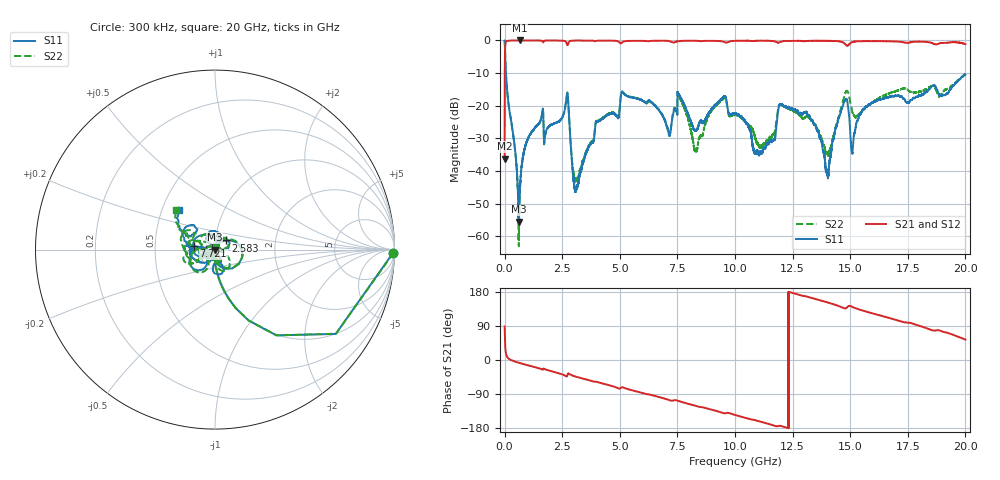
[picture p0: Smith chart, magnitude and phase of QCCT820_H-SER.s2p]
!{QCCT820}
!Johanson Technology Inc.
!www.johansontechnology.com
!Test Board Conditions:
!Substrate Type  RO4350B
!Substrate Thickness  20 mil
!Substrate Dk  3.66
!TL Type: GCPW
!TL Trace Width  34 mil
!TL Gap  10 mil
!Electrode orientation  Horizontal
!DUT TOPOLOGY	SERIES
!Mounting Pad LxW  26x52 mil
! Created Sat Jan  9 19:21:07 2021
# hz S ma R 50
! 2 Port Network Data from SP1.SP block
! freq  magS11  angS11  magS21  angS21  magS12  angS12  magS22  angS22
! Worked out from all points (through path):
!   20001 points, 300 kHz to 20 GHz, reference 50 ohm
!   highest |S21| = 0.00 dB at 661.3 MHz (marker M1); lowest = -36.2 dB at 300 kHz (marker M2)
!   group delay of S21, straight-line fit = 42 ps
!   lowest |S11| = -55.6 dB at 616.3 MHz (marker M3), VSWR 1.00, Z = 49.8 + j0.028 ohm
!   |S11| at or under -10 dB: 57.01 MHz to end of sweep
!   |S22| runs from -63.0 to 0.0 dB; largest |S21 - S12| = 0.015
!   S11 on the Smith chart (normalised r, x): 300 kHz: open; 2.583 GHz: 1.12, +0.12; 7.721 GHz: 0.79, +0.03; 20 GHz: 0.61, +0.30
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300000  0.9935 -0.9  0.01552 88.4  0.01569 89.2  0.9945 -1.0
1.113e8  0.1658 -82.3  0.9851 8.2  0.9851 8.1  0.1665 -82.1
6.163e8  0.001668 170.3  0.9989 -7.3  0.9988 -7.3  0.0007043 -161.2
6.613e8  0.004868 99.8  0.9995 -8.1  0.9977 -8.1  0.004485 90.4
1.1063e9  0.03639 77.6  0.9988 -15.5  0.9983 -15.5  0.03631 73.8
2.5833e9  0.07857 40.5  0.9843 -39.9  0.9856 -39.8  0.07863 45.1
2.7443e9  0.1404 -48.7  0.8591 -36.7  0.8591 -36.7  0.1416 -44.7
3.0543e9  0.005208 -132.3  0.9961 -43.2  0.9961 -43.2  0.007195 -86.5
3.3343e9  0.01071 -160.5  0.9977 -48.0  0.9977 -48.0  0.01145 -105.8
5.1313e9  0.1597 -152.4  0.949 -72.3  0.9481 -72.2  0.1612 -146.3
6.6673e9  0.08934 171.4  0.9897 -97.2  0.9891 -97.1  0.08814 178.0
7.7213e9  0.1182 171.2  0.9842 -111.4  0.985 -111.4  0.1063 153.1
8.2913e9  0.04211 -130.0  0.9888 -121.0  0.9881 -120.9  0.02083 56.8
1.00003e10  0.07586 -66.3  0.9862 -145.0  0.9879 -144.9  0.07212 -58.9
1.10863e10  0.01985 13.3  0.9901 -162.4  0.9894 -162.4  0.023 -163.0
1.19923e10  0.1047 96.5  0.956 -174.1  0.9559 -174.0  0.1052 128.5
1.33343e10  0.06069 62.7  0.9858 163.6  0.9863 163.6  0.05838 90.2
1.40083e10  0.00927 -25.6  0.9844 151.9  0.9827 152.1  0.01852 143.8
1.47713e10  0.1215 -177.4  0.8875 136.3  0.8865 136.2  0.15 -161.0
1.51013e10  0.01958 -38.7  0.9464 140.0  0.9474 140.3  0.07802 158.2
1.66673e10  0.1348 -164.4  0.973 111.2  0.9645 111.3  0.1537 -148.9
2e10  0.2991 131.5  0.8766 53.9  0.867 53.8  0.3085 134.3
